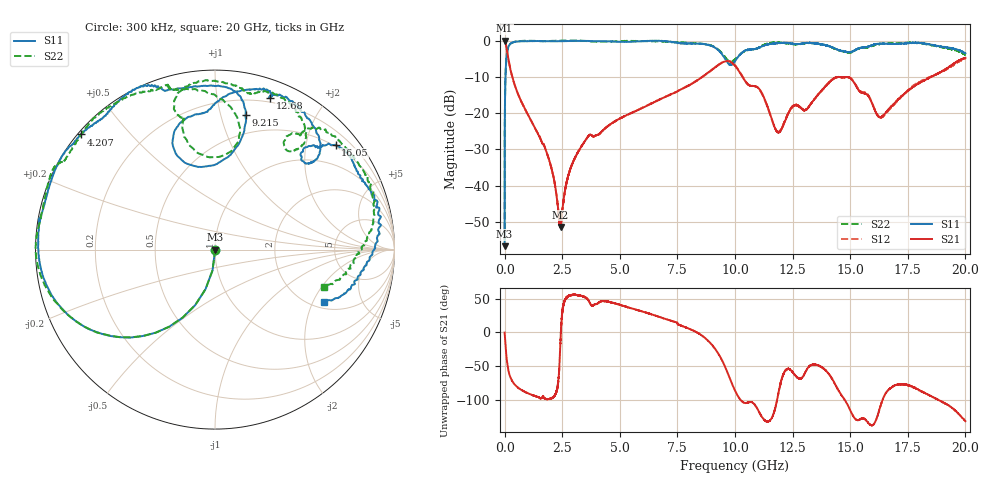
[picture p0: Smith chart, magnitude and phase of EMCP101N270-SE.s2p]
!EMCP101N270
!Johanson Technology Inc.
!www.johansontechnology.com
!Test Board Conditions:
!Substrate Type  RO4350B
!Substrate Thickness  10 mil
!Substrate Dk  3.66
!TL Type: GCPW
!TL Trace Width  20 mil
!TL Gap  10 mil
!PART MODE SINGLE ENDED (AKA BYPASS)
!DUT TOPOLOGY	SERIES-SHUNT
# MHz S  dB  R 50
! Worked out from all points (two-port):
!   20001 points, 300 kHz to 20 GHz, reference 50 ohm
!   highest |S21| = 0.00 dB at 1.3 MHz (marker M1); lowest = -51.5 dB at 2.428 GHz (marker M2)
!   |S21| within 3 dB of the highest: start of sweep to 111.1 MHz
!   lowest |S11| = -56.7 dB at 300 kHz (marker M3), VSWR 1.00, Z = 50.1 - j0.128 ohm
!   |S11| at or under -10 dB: start of sweep to 37.62 MHz
!   |S22| runs from -55.0 to 0.1 dB; largest |S21 - S12| = 0.026
!   S11 on the Smith chart (normalised r, x): 300 kHz: 1.00, -0.00; 4.207 GHz: 0.01, +0.37; 9.215 GHz: 0.33, +1.20; 12.68 GHz: 0.16, +1.41; 16.05 GHz: 0.47, +2.61; 20 GHz: 2.30, -2.44
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0.3  -56.73 -61.7  -0.01 -0.2  -0.00 -0.2  -55.01 -55.6
1.3  -38.88 -89.8  -0.00 -0.7  -0.00 -0.7  -38.83 -90.1
103.298  -3.42 -133.5  -2.70 -43.1  -2.68 -43.1  -3.46 -133.3
205.297  -1.18 -153.1  -6.47 -62.1  -6.44 -62.2  -1.21 -152.6
626.291  -0.19 -175.5  -15.38 -83.3  -15.39 -83.6  -0.12 -173.2
1866.272  -0.13 167.8  -31.66 -99.4  -31.59 -99.3  -0.09 163.5
2428.264  -0.12 161.3  -51.46 -10.6  -51.38 -11.1  0.03 156.7
2790.258  -0.08 156.5  -36.69 54.3  -36.68 53.8  0.06 154.1
3334.25  -0.02 149.0  -29.18 54.2  -29.21 54.2  -0.00 151.6
4207.237  -0.13 139.4  -25.11 46.4  -25.13 46.2  -0.22 147.1
6667.2  -0.02 114.6  -16.43 23.6  -16.39 23.2  -0.19 118.9
9215.162  -2.30 77.2  -6.99 -28.4  -7.00 -27.7  -2.15 82.6
10000.15  -5.67 109.8  -6.91 -86.6  -6.79 -86.2  -5.12 100.8
11107.13  -1.72 89.6  -13.79 -122.2  -13.89 -123.0  -1.65 105.9
11842.12  -0.68 74.7  -25.13 -97.5  -25.17 -96.4  -0.53 91.7
12676.11  -0.93 70.0  -17.81 -66.2  -17.69 -66.4  -0.99 77.4
13334.1  -0.65 63.1  -17.08 -48.3  -17.03 -48.8  -0.69 66.4
14872.08  -3.13 43.5  -10.03 -106.8  -10.05 -105.7  -3.23 52.5
16048.06  -1.02 40.9  -18.83 -135.5  -18.77 -137.2  -1.21 51.4
16667.05  -0.86 30.7  -18.93 -85.3  -19.25 -85.2  -0.74 41.9
18152.03  -0.78 6.8  -11.14 -88.7  -10.97 -89.0  -0.83 13.2
20000  -3.43 -25.5  -4.75 -132.1  -4.82 -129.8  -3.84 -18.8
